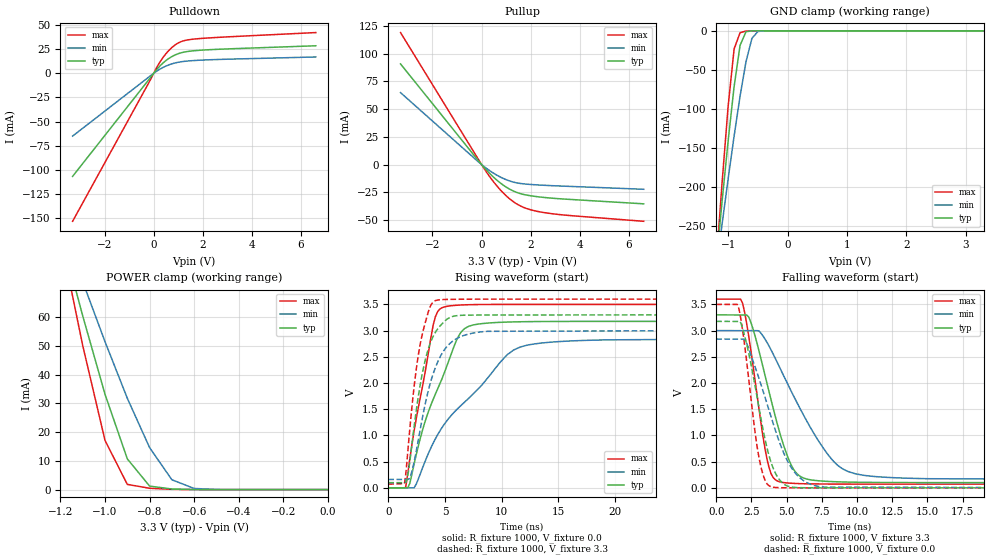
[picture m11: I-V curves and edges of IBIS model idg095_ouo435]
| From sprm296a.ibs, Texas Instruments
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[Model]   idg095_ouo435
Model_type   I/O
Vinh = 2.00
Vinl = 0.80
Enable   Active-Low
Polarity   Non-Inverting
| signals   A, GZ, Y
Vmeas = 1.5
|   typ   min   max
C_comp   4.049p   4.002p   4.089p
|   typ   min   max
[Temperature Range]   25   -40   125
|   typ   min   max
[Voltage Range]   3.30V   3.00V   3.60V
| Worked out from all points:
|   slope of the pulldown table from 0 to 0.495 V, typ, clamps not added: 37.7 ohm
|   slope of the pullup table from 0 to 0.495 V, typ, clamps not added: 42.7 ohm
|   GND clamp passes 1 mA (typ) near -0.69 V on its own axis
|   POWER clamp passes 1 mA (typ) near -0.78 V on its own axis
|   rising waveform, R_fixture 1000, V_fixture 0.0: 20-80 % time 3.06ns typ, 6.04ns min, 1.71ns max; typ from 0 V to 3.18 V
|   falling waveform, R_fixture 1000, V_fixture 3.3: 20-80 % time 1.89ns typ, 3.42ns min, 1.14ns max; typ from 3.3 V to 0.099 V
|   rising waveform, R_fixture 1000, V_fixture 3.3: 20-80 % time 1.51ns typ, 1.93ns min, 1.21ns max; typ from 0.099 V to 3.3 V
|   falling waveform, R_fixture 1000, V_fixture 0.0: 20-80 % time 1.4ns typ, 2.15ns min, 977ps max; typ from 3.18 V to 0 V
[Pulldown]
|   Voltage   I(typ)   I(min)   I(max)
-3.3V     -106.6mA   -64.96mA   -153.1mA
-200mV    -6.638mA   -3.888mA   -9.861mA
200mV     6.136mA    3.487mA    9.379mA
500mV     13.23mA    7.514mA    20.3mA
800mV     18.12mA    10.25mA    27.98mA
1V        20.32mA    11.45mA    31.43mA
1.2V      21.76mA    12.24mA    33.52mA
1.7V      23.5mA     13.33mA    35.59mA
6.6V      28.52mA    16.93mA    42.18mA
[GND_clamp]
|   Voltage   I(typ)   I(min)   I(max)
-3.3V     -2.096A    -1.605A    -2.685A
-1.2V     -296.1mA   -304.5mA   -296.4mA
-1.1V     -216.7mA   -246.3mA   -192.3mA
-1V       -140.7mA   -189.5mA   -96.19mA
-900mV    -71.48mA   -134.8mA   -23.23mA
-800mV    -18.7mA    -83.78mA   -2.443mA
-700mV    -1.136mA   -39.52mA   -238.9uA
-600mV    -46.29uA   -9.639mA   -13.6uA
-500mV    -2.239uA   -853.4uA   -473.2nA
-300mV    -4.174nA   -2.864uA   -494pA
3.3V      266.4pA    359.3nA    310.9pA
[Pullup]
|   Voltage   I(typ)   I(min)   I(max)
-3.3V     90.83mA    64.92mA    119.1mA
100mV     -2.569mA   -1.78mA    -3.482mA
400mV     -9.588mA   -6.59mA    -13.07mA
700mV     -15.54mA   -10.57mA   -21.33mA
1.2V      -22.92mA   -15.27mA   -32mA
1.7V      -26.98mA   -17.44mA   -38.62mA
2V        -28.23mA   -18.01mA   -40.89mA
2.5V      -29.63mA   -18.7mA    -43.25mA
3.5V      -31.38mA   -19.67mA   -45.9mA
6.6V      -35.51mA   -22.36mA   -51.28mA
[POWER_clamp]
|   Voltage   I(typ)   I(min)   I(max)
-3.3V     758.3mA    581mA      973mA
-1.2V     89.56mA    93.92mA    87.99mA
-1.1V     60.47mA    72.37mA    50.13mA
-1V       33.18mA    51.49mA    17.12mA
-900mV    10.7mA     31.81mA    1.812mA
-800mV    1.221mA    14.62mA    465.8uA
-700mV    206.6uA    3.422mA    95.32uA
-600mV    31.41uA    399uA      7.822uA
-500mV    2.639uA    43.56uA    300.9nA
0V        1pA        1pA        1pA
[Ramp]
|   I(typ)   I(min)   I(max)
dV/dt_r   1.905/3.062n   1.702/6.039n   2.100/1.708n
dV/dt_f   1.920/1.887n   1.704/3.423n   2.118/1.136n
[Rising Waveform]
R_fixture = 1000
V_fixture = 0.0
|  pu_on
|  TIME   V(typ)   V(min)   V(max)
0s        6nV        15nV       4nV
1.523ns   415.6uV    816.4uV    7.923mV
1.896ns   87.54mV    816.4uV    560mV
2.27ns    455.3mV    816.4uV    1.085V
3.95ns    1.688V     853.2mV    3.103V
4.697ns   2.064V     1.139V     3.433V
6.003ns   2.812V     1.488V     3.483V
6.75ns    3.043V     1.641V     3.491V
11.79ns   3.169V     2.696V     3.499V
30ns      3.176V     2.837V     3.499V
[Falling Waveform]
R_fixture = 1000
V_fixture = 3.3
V_fixture_min = 3.0
V_fixture_max = 3.6
|  pd_on
|  TIME   V(typ)   V(min)   V(max)
0s        3.3V       3V         3.6V
1.872ns   3.298V     2.999V     3.52V
2.448ns   3.163V     2.999V     2.637V
3.456ns   2.154V     2.841V     754.2mV
3.888ns   1.684V     2.634V     273.6mV
4.319ns   1.235V     2.4V       133.8mV
5.903ns   230.7mV    1.539V     81.1mV
7.918ns   123.4mV    640.9mV    72.94mV
9.357ns   110.2mV    312.2mV    71.51mV
30ns      99.39mV    159.9mV    70.79mV
[Rising Waveform]
R_fixture = 1000
V_fixture = 3.3
V_fixture_min = 3.0
V_fixture_max = 3.6
|  pd_off
|  TIME   V(typ)   V(min)   V(max)
0s        99.39mV    159.8mV    70.79mV
1.415ns   99.39mV    160.6mV    81.03mV
1.643ns   162.4mV    160.6mV    514.5mV
1.947ns   597.3mV    220.8mV    1.253V
2.707ns   1.833V     995.1mV    2.618V
3.542ns   2.664V     1.873V     3.37V
4.074ns   2.94V      2.251V     3.563V
5.517ns   3.258V     2.771V     3.596V
8.024ns   3.297V     2.971V     3.599V
30ns      3.3V       3V         3.6V
[Falling Waveform]
R_fixture = 1000
V_fixture = 0.0
|  pu_off
|  TIME   V(typ)   V(min)   V(max)
0s        3.176V     2.838V     3.499V
1.561ns   3.175V     2.837V     3.466V
2.154ns   2.748V     2.765V     2.418V
3.012ns   1.56V      2.105V     611.1mV
3.408ns   997.9mV    1.774V     183.3mV
3.87ns    504.5mV    1.375V     23.83mV
4.53ns    142.4mV    841.8mV    3.267mV
5.322ns   17.04mV    388.8mV    1.145mV
7.169ns   1.083mV    32.49mV    229.3uV
30ns      1.252uV    5.102uV    682.8nV
